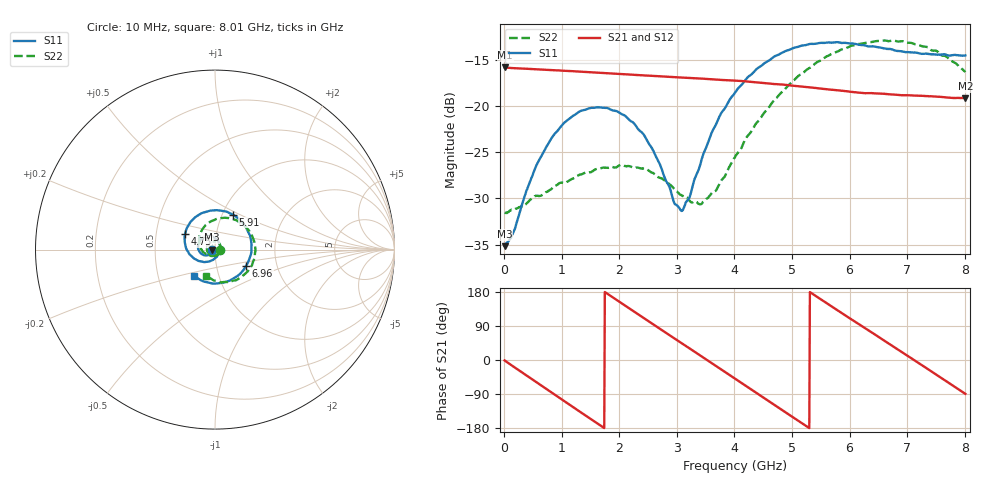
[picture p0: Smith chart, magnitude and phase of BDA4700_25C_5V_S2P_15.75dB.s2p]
!Agilent Technologies,E5071B,MY42404982,A.09.10
!Date: Mon Oct 20 13:34:07 2025
!Data & Calibration Information:
!Freq	S11:SOLT2(ON)	S21:SOLT2(ON)	S12:SOLT2(ON)	S22:SOLT2(ON)
# Hz S RI R 50
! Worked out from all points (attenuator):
!   801 points, 10 MHz to 8.01 GHz, reference 50 ohm
!   highest |S21| = -15.85 dB at 20 MHz (marker M1); lowest = -19.2 dB at 8.01 GHz (marker M2)
!   lowest |S11| = -35.2 dB at 10 MHz (marker M3), VSWR 1.04, Z = 48.3 - j0.104 ohm
!   |S11| at or under -10 dB: start of sweep to end of sweep
!   |S22| runs from -31.6 to -12.9 dB; largest |S21 - S12| = 0.0012
!   S11 on the Smith chart (normalised r, x): 10 MHz: 0.97, -0.00; 4.75 GHz: 0.70, +0.13; 5.91 GHz: 1.12, +0.46; 6.96 GHz: 1.39, -0.27; 8.01 GHz: 0.76, -0.23
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1e7  -0.0174 -0.00108  0.1612 -0.00349  0.1612 -0.0037  0.0265 -0.00104
2e7  -0.0178 -0.00175  0.1611 -0.00626  0.1611 -0.00675  0.0264 -0.00124
1.6e8  -0.0183 -0.00955  0.1529 -0.0468  0.1529 -0.0469  0.0264 -0.00788
5.1e8  -0.0332 -0.0281  0.0943 -0.1268  0.0941 -0.1268  0.0163 -0.0277
7.4e8  -0.0512 -0.0322  0.0349 -0.1526  0.0349 -0.1527  0.00174 -0.0343
1.35e9  -0.0943 0.00542  -0.1167 -0.0988  -0.1168 -0.0989  -0.04 -0.015
1.72e9  -0.0855 0.0469  -0.1506 -0.00629  -0.1506 -0.00629  -0.0436 0.0158
2.09e9  -0.0501 0.0734  -0.1211 0.0856  -0.1212 0.0857  -0.0243 0.0407
2.42e9  -0.00835 0.0698  -0.053 0.1361  -0.0531 0.1362  0.00425 0.0456
2.68e9  0.0174 0.047  0.0125 0.1441  0.0125 0.1441  0.0226 0.0344
2.96e9  0.028 0.00984  0.0781 0.1195  0.0782 0.1194  0.0324 0.0144
3.1e9  0.0253 -0.0101  0.1047 0.0962  0.1043 0.0965  0.0327 0.00147
3.44e9  -0.00456 -0.0523  0.1388 0.0205  0.1389 0.0205  0.0161 -0.0251
3.75e9  -0.0554 -0.0694  0.1274 -0.0536  0.1275 -0.0537  -0.0138 -0.036
4.01e9  -0.1029 -0.0573  0.0895 -0.1035  0.0896 -0.1035  -0.0436 -0.0298
4.75e9  -0.1668 0.0868  -0.0736 -0.1082  -0.0733 -0.1086  -0.0875 0.0702
5.35e9  -0.0648 0.2063  -0.125 0.0104  -0.1252 0.0101  -0.0079 0.1631
5.91e9  0.0989 0.1952  -0.0586 0.1051  -0.0589 0.1048  0.129 0.1577
6.68e9  0.2024 -0.00973  0.0841 0.0792  0.0844 0.0791  0.2227 -0.0218
6.96e9  0.1722 -0.0926  0.1099 0.031  0.11 0.0305  0.2 -0.0959
7.49e9  0.0364 -0.186  0.0894 -0.068  0.0894 -0.0681  0.0808 -0.1819
8.01e9  -0.1158 -0.1473  0.00123 -0.1101  0.00141 -0.1102  -0.0477 -0.1445
